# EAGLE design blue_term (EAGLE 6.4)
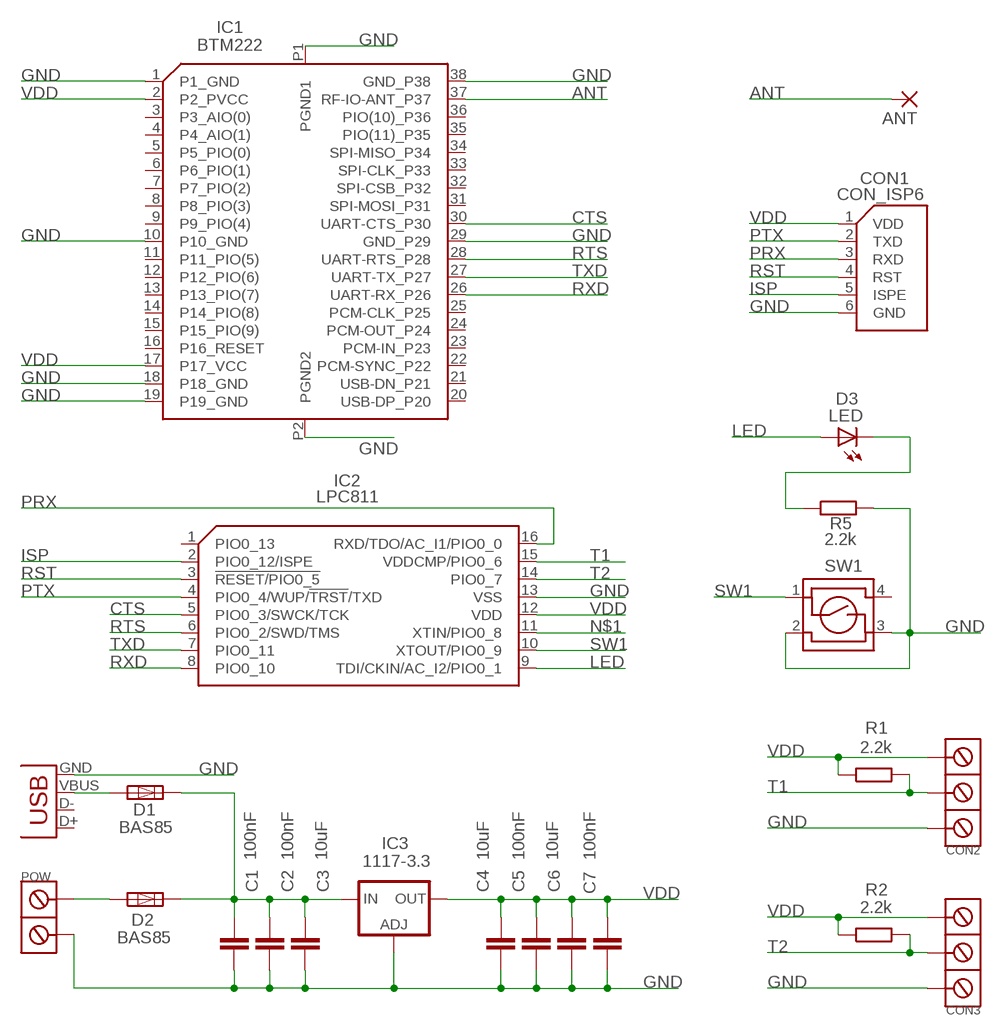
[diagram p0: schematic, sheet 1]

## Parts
ANT  2,54/1,0  [2,54/1,0]
C1  100nF  C-EUC1206  [C1206]
C2  100nF  C-EUC1206  [C1206]
C3  10uF  C-EUC1206  [C1206]
C4  10uF  C-EUC1206  [C1206]
C5  100nF  C-EUC1206  [C1206]
C6  10uF  C-EUC1206  [C1206]
C7  100nF  C-EUC1206  [C1206]
CON1  CON_ISP6  [CON6]
CON2  ARK3ARK3/500  [ARK3/500]
CON3  ARK3ARK3/500  [ARK3/500]
D1  BAS85  R-EU_R1206  [R1206]
D2  BAS85  R-EU_R1206  [R1206]
D3  LED  LEDCHIPLED_1206  [CHIPLED_1206]
IC1  BTM222  [BTM222]
IC2  LPC811  [TSSOP16]
IC3  1117-3.3  LM317MABDT  [DPACK]
POW  ARK2ARK2/500  [ARK2/500]
R1  2.2k  R-EU_R1206  [R1206]
R2  2.2k  R-EU_R1206  [R1206]
R5  2.2k  R-EU_R1206  [R1206]
SW1  6X6  [6X6]
USB  USB-MICROB  [USB-MICROB]

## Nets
ANT: ANT.1(P) IC1.37(RF-IO-ANT_P37)
CTS: IC1.30(UART-CTS_P30) IC2.5(PIO0_3/SWCK/TCK)
GND: C1.2 C2.2 C3.2 C4.2 C5.2 C6.2 C7.2 CON1.6(GND) CON2.1 CON3.1 IC1.1(P1_GND) IC1.10(P10_GND) IC1.18(P18_GND) IC1.19(P19_GND) IC1.29(GND_P29) IC1.38(GND_P38) IC1.P1(PGND1) IC1.P2(PGND2) IC2.13(VSS) IC3.1(ADJ) POW.2 R5.2 SW1.2 SW1.3 USB.GND
ISP: CON1.5(ISPE) IC2.2(PIO0_12/ISPE)
LED: D3.A IC2.9(TDI/CKIN/AC_I2/PIO0_1)
N$1: IC2.11(XTIN/PIO0_8)
N$2: D3.C R5.1
N$10: D1.1 USB.VBUS
N$11: C1.1 C2.1 C3.1 D1.2 D2.2 IC3.3(IN)
N$12: D2.1 POW.1
PRX: CON1.3(RXD) IC2.16(RXD/TDO/AC_I1/PIO0_0)
PTX: CON1.2(TXD) IC2.4(PIO0_4/WUP/!TRST!/TXD)
RST: CON1.4(RST) IC2.3(!RESET/PIO0_5)
RTS: IC1.28(UART-RTS_P28) IC2.6(PIO0_2/SWD/TMS)
RXD: IC1.26(UART-RX_P26) IC2.8(PIO0_10)
SW1: IC2.10(XTOUT/PIO0_9) SW1.1
T1: CON2.2 IC2.15(VDDCMP/PIO0_6) R1.2
T2: CON3.2 IC2.14(PIO0_7) R2.2
TXD: IC1.27(UART-TX_P27) IC2.7(PIO0_11)
VDD: C4.1 C5.1 C6.1 C7.1 CON1.1(VDD) CON2.3 CON3.3 IC1.2(P2_PVCC) IC1.17(P17_VCC) IC2.12(VDD) IC3.4(OUT) R1.1 R2.1
Unconnected: IC1.3(P3_AIO(0)) IC1.4(P4_AIO(1)) IC1.5(P5_PIO(0)) IC1.6(P6_PIO(1)) IC1.7(P7_PIO(2)) IC1.8(P8_PIO(3)) IC1.9(P9_PIO(4)) IC1.11(P11_PIO(5)) IC1.12(P12_PIO(6)) IC1.13(P13_PIO(7)) IC1.14(P14_PIO(8)) IC1.15(P15_PIO(9)) IC1.16(P16_RESET) IC1.20(USB-DP_P20) IC1.21(USB-DN_P21) IC1.22(PCM-SYNC_P22) IC1.23(PCM-IN_P23) IC1.24(PCM-OUT_P24) IC1.25(PCM-CLK_P25) IC1.31(SPI-MOSI_P31) IC1.32(SPI-CSB_P32) IC1.33(SPI-CLK_P33) IC1.34(SPI-MISO_P34) IC1.35(PIO(11)_P35) IC1.36(PIO(10)_P36) IC2.1(PIO0_13) SW1.4 USB.D+ USB.D-

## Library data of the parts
ANT = wirepad:2,54/1,0: THROUGH-HOLE PAD
C1-C7 = rcl:C-EU: CAPACITOR, European symbol
CON1 = LPC1114:CON_ISP6
CON2 CON3 = dimmer:ARK3
D1 D2 R1 R2 R5 = rcl:R-EU_: RESISTOR, European symbol
D3 = led:LED: LED
IC1 = BTM222:BTM222
IC2 = LPC8xx:LPC811
IC3 = v-reg:LM317?*: 500 mA Adjustable Output Positive Voltage Regulator Source: http://www.onsemi.co.jp .. LM317M-D.PDF
POW = dimmer:ARK2
SW1 = sw:6X6
USB = SparkFun:USB: USB Connectors USB-B-PTH is fully proven SKU : PRT-00139 USB-miniB is fully proven SKU : PRT-00587 USB-A-PCB is untested. USB-A-H is throughly reviewed, but untested. Spark Fun Electronics SKU : PRT-00437 USB-B-SMT is throughly reviewed, but untested. Needs silkscreen touching up. USB-A-S has not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

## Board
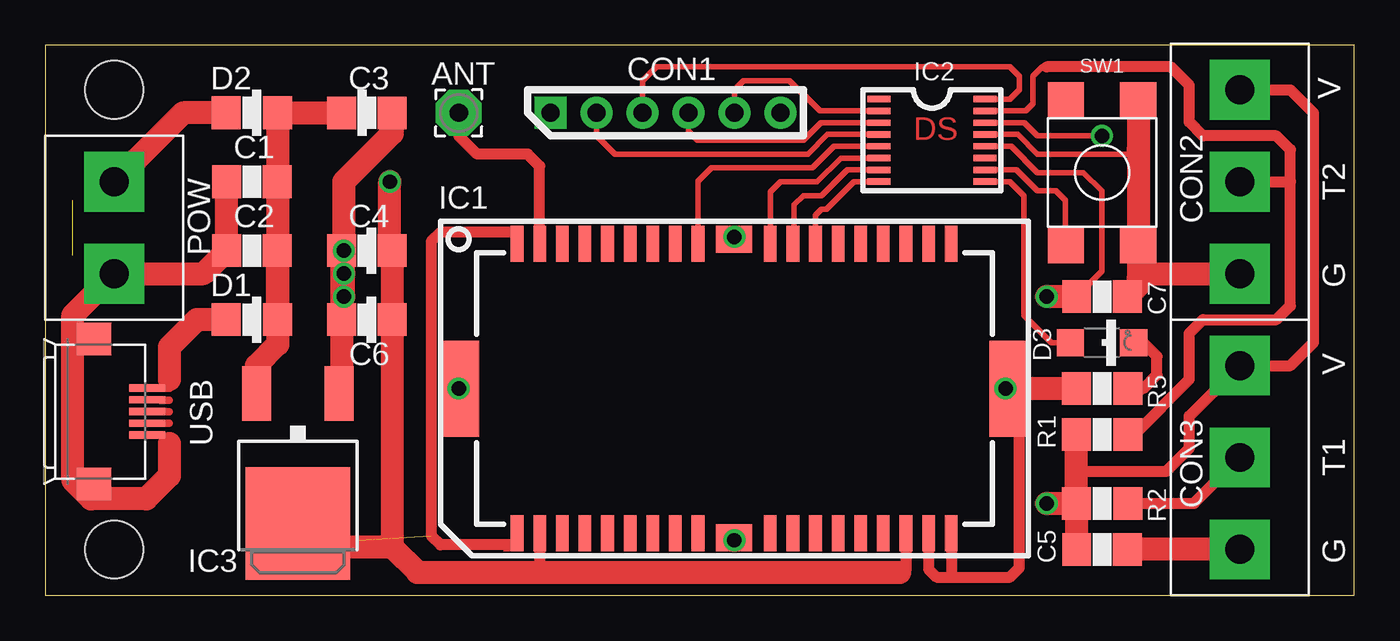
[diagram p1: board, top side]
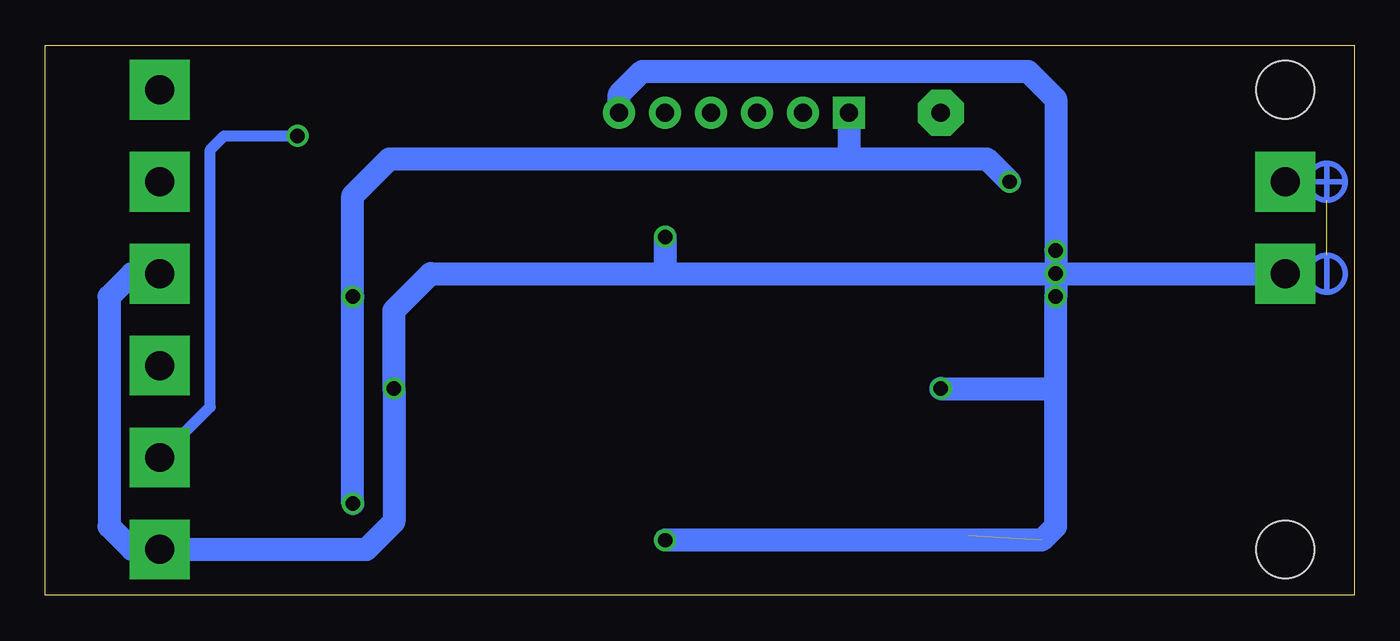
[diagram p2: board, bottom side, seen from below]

Size 72.37 x 30.4 mm. Coordinates in mm from the lower left corner, seen from the top.
Outline: 0,0 72.37,0 72.37,30.4 0,30.4 0,0
Copper layers (1*16): Top 0.035mm / dielectric 1.5mm / Bottom 0.035mm
Design rules "default": minimum track width 10mil, minimum drill 24mil, track to track 8mil, track to pad 8mil, pad to pad 8mil, via to via 8mil, smd to smd 8mil, copper to edge 40mil, drill to drill 8mil, minimum pad ring 10mil, minimum via ring 8mil, stop-mask expansion 4mil, vias tented up to drill 0mil, thermal gap 10mil
Holes 3.2 mm at 3.81,27.94 3.81,2.54

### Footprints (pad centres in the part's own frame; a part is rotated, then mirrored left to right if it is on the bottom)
2,54/1,0 = drill 1.016 pad 2.54 octagon: 1 0,0
C1206 = smd 1.6 x 1.8: 1 -1.4,0; 2 1.4,0
CON6 = drill 1 pad 1.778 square: 1 0,6.35 | drill 1 pad 1.778: 2 0,3.81; 3 0,1.27; 4 0,-1.27; 5 0,-3.81; 6 0,-6.35
ARK3/500 = drill 1.6 pad 3.302 square: 1 -5.08,0; 2 0,0; 3 5.08,0
R1206 = smd 1.6 x 1.803: 1 -1.422,0; 2 1.422,0
CHIPLED_1206 = smd 1.5 x 1.5: A 0,-1.75; C 0,1.75
BTM222 = smd 0.7 x 2: 1 -12.015,-8; 2 -10.765,-8; 3 -9.515,-8; 4 -8.265,-8; 5 -7.015,-8; 6 -5.765,-8; 7 -4.515,-8; 8 -3.265,-8; 9 -2.015,-8; 11 1.985,-8; 12 3.235,-8; 13 4.485,-8; 14 5.735,-8; 15 6.985,-8; 16 8.235,-8; 17 9.485,-8; 18 10.735,-8; 19 11.985,-8; 20 11.985,8; 21 10.735,8; 22 9.485,8; 23 8.235,8; 24 6.985,8; 25 5.735,8; 26 4.485,8; 27 3.235,8; 28 1.985,8; 30 -2.015,8; 31 -3.265,8; 32 -4.515,8; 33 -5.765,8; 34 -7.015,8; 35 -8.265,8; 36 -9.515,8; 37 -10.765,8; 38 -12.015,8 | smd 2 x 1.5: 10 -0.015,-8.25; 29 -0.015,8.25 | smd 2 x 5.3: P1 -15.115,0; P2 15.085,0
TSSOP16 = smd 0.356 x 1.27: 1 -2.275,-2.918; 2 -1.625,-2.918; 3 -0.975,-2.918; 4 -0.325,-2.918; 5 0.325,-2.918; 6 0.975,-2.918; 7 1.625,-2.918; 8 2.275,-2.918; 9 2.275,2.918; 10 1.625,2.918; 11 0.975,2.918; 12 0.325,2.918; 13 -0.325,2.918; 14 -0.975,2.918; 15 -1.625,2.918; 16 -2.275,2.918
DPACK = smd 1.6 x 3: 1 -2.28,-4.8; 3 2.28,-4.8 | smd 5.8 x 6.2: 4 0,2.38
ARK2/500 = drill 1.6 pad 3.302 square: 1 -2.54,0; 2 2.54,0
6X6 = smd 2 x 2: 1 -4,2; 2 -4,-2; 3 4,-2; 4 4,2
USB-MICROB = smd 0.4 x 2: D+ 0,3.1; D- -0.65,3.1; GND 1.3,3.1; ID 0.65,3.1; VBUS -1.3,3.1 | smd 1.8 x 1.9: GND@2 -4,0.15; GND@3 4,0.15

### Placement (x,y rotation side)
ANT  22.86,26.67 0 top
C1  11.43,22.86 180 top
C2  11.43,19.05 180 top
C3  17.78,26.67 0 top
C4  17.78,19.05 180 top
C5  58.42,2.54 0 top
C6  17.78,15.24 180 top
C7  58.42,16.51 0 top
CON1  34.29,26.67 90 top
CON2  66.04,22.86 90 top
CON3  66.04,7.62 90 top
D1  11.43,15.24 0 top
D2  11.43,26.67 0 top
D3  58.42,13.97 270 top
IC1  38.1,11.43 0 top
IC2  49.02,25.15 270 top
IC3  13.97,6.35 180 top
POW  3.81,20.32 270 top
R1  58.42,8.89 0 top
R2  58.42,5.08 0 top
R5  58.42,11.43 180 top
SW1  58.42,23.37 90 top
USB  2.54,10.16 270 top

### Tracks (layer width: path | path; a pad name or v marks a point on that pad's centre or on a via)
ANT
  Top 0.61: IC1.37 27.34,23.72 26.67,24.38 23.88,24.38 22.86,25.4 ANT.1
CTS
  Top 0.305: IC1.30 36.09,22.88 36.83,23.62 42.42,23.62 43.62,24.82 IC2.5
GND  (via drill 0.8)  (1 unrouted)
  Top 0.305: USB.GND 6.83,8.86 6.86,8.89 6.86,8.38 | IC2.13 53.78,25.47 54.86,24.38 60.17,24.38 60.42,24.64
  Top 0.61: IC1.38 26.09,19.99 26.16,20.07 21.84,20.07 21.34,19.56 21.34,3.3 21.84,2.79 25.91,2.79 26.09,2.97 IC1.1 | IC1.18 48.84,1.46 49.28,1.02 50.29,1.02 | 50.29,1.02 53.34,1.02 53.85,1.52 53.85,10.77 IC1.P2 | IC1.19 50.09,1.22 50.29,1.02
  Top 1.27: C4.2 C6.2 16.38,11.28 IC3.1 | C1.2 C2.2 8.76,17.78 POW.2 1.52,15.49 1.52,6.35 2.54,5.33 5.59,5.33 6.86,6.6 6.86,8.38 | v16.51,19.05 C4.2 | CON3.1 C5.2 | C3.2 19.18,25.53 16.51,22.86 v16.51,19.05 | SW1.3 60.42,24.64 SW1.2 60.42,17.53 | 60.42,17.53 60.42,17.11 C7.2 | 60.42,17.53 60.67,17.78 CON2.1 | R5.2 IC1.P2 v53.09,11.43 | v16.51,16.51 v16.51,17.78 v16.51,19.05 | v16.51,19.05 16.51,19.18 C4.2 | IC1.29 38.09,19.8 v38.1,19.81 | IC1.10 38.09,3.03 v38.1,3.05 | IC1.P1 v22.86,11.43
  Bottom 1.27: CON2.1 67.56,17.78 68.83,16.51 68.83,3.81 67.56,2.54 CON3.1 54.61,2.54 53.09,4.06 v53.09,11.43 53.09,15.75 51.05,17.78 37.85,17.78 | 37.85,17.78 v16.51,17.78 | CON1.6 40.64,27.69 39.37,28.96 18.03,28.96 16.51,27.43 v16.51,19.05 v16.51,17.78 | v16.51,17.78 POW.2 | v16.51,17.78 v16.51,16.51 16.51,11.68 | v38.1,19.81 38.1,18.03 37.85,17.78 | 16.51,11.68 16.51,3.81 17.27,3.05 v38.1,3.05 | v22.86,11.43 16.76,11.43 16.51,11.68
ISP
  Top 0.305: IC2.2 42.83,26.77 41.15,28.45 38.61,28.45 38.1,27.94 CON1.5
LED
  Top 0.305: 56.39,13.97 55.63,13.97 54.1,15.49 54.1,22.1 53.34,22.86 51.95,22.86 IC2.9
  Top 0.61: D3.A 56.39,13.97
N$2
  Top 0.61: R5.1 60.71,11.43 61.47,12.19 61.47,13.21 60.71,13.97 D3.C
N$3
  Top 0.406: 6.35,10.79 6.86,10.79
N$4
  Top 0.406: 6.48,10.16 6.86,10.16
N$5
  Top 0.406: 6.35,9.52 6.86,9.52
N$6  (1 unrouted)
  Bottom 0.305: 1.52,23.88 1.52,21.84 | 1.52,18.8 1.52,16.76
N$7
  Bottom 0.305: 0.51,22.86 2.54,22.86
N$10
  Top 0.305: 6.89,11.46 6.89,12.67 6.86,11.94
  Top 0.406: USB.VBUS 6.89,11.46
  Top 1.27: D1.1 8.38,15.24 6.86,13.72 6.86,11.94
N$11
  Top 1.27: 12.85,22.86 D2.2 C3.1 | 12.85,22.86 12.85,19.05 | 12.85,19.05 D1.2 | C1.1 12.85,22.86 | 12.85,19.05 C2.1 12.83,15.26 D1.2 | D1.2 12.85,13.87 11.68,12.7 IC3.3
N$12
  Top 1.27: D2.1 7.62,26.67 POW.1
PRX
  Top 0.305: IC2.16 53.33,27.42 53.85,27.94 53.85,28.7 53.34,29.21 33.78,29.21 33.02,28.45 CON1.3
PTX
  Top 0.305: IC2.4 43.25,25.47 42.16,24.38 31.5,24.38 30.48,25.4 CON1.2
RST
  Top 0.305: IC2.3 42.88,26.12 41.91,25.15 36.07,25.15 35.56,25.65 CON1.4
RTS
  Top 0.305: IC1.28 40.09,22.31 40.64,22.86 42.67,22.86 43.98,24.17 IC2.6
RXD
  Top 0.305: IC2.8 44.72,22.87 43.18,21.34 42.93,21.34 42.59,21 IC1.26
SW1
  Top 0.305: IC2.10 53.7,23.52 54.86,22.35 55.88,22.35 56.39,21.84 56.39,19.4 SW1.1
T1
  Top 0.305: 55.37,29.21 55.12,29.21 54.61,28.7 54.61,27.18 54.2,26.77 IC2.15
  Top 0.61: 55.37,29.21 62.23,29.21 63.25,28.19 63.25,26.16 64.01,25.4 68.07,25.4 68.83,24.64 68.83,22.86 | R1.2 60.2,8.89 63.25,11.94 63.25,14.48 64.01,15.24 68.07,15.24 68.83,16 68.83,22.86 | CON2.2 68.83,22.86
T2  (via drill 0.8)
  Top 0.305: IC2.14 54.14,26.12 54.86,25.4 v58.42,25.4
  Top 0.61: R2.2 63.5,5.08 CON3.2
  Bottom 0.61: CON3.2 63.25,10.41 63.25,24.64 62.48,25.4 v58.42,25.4
TXD
  Top 0.305: IC2.7 44.35,23.52 42.93,22.1 41.91,22.1 41.4,21.59 41.4,19.5 IC1.27
VDD  (via drill 0.8)
  Top 0.305: IC2.12 53.41,24.82 54.86,23.37 57.4,23.37 58.42,22.35 58.42,17.91 C7.1
  Top 0.61: IC1.2 27.34,1.37 27.43,1.27 | IC1.17 47.59,1.44 47.24,1.27 | 57,6.86 61.98,6.86 63.25,8.13 63.25,9.91 CON3.3 68.83,12.7 70.1,13.97 70.1,26.67 68.83,27.94 CON2.3
  Top 1.27: 19.18,2.66 C6.1 19.18,18.92 | 19.18,2.66 20.57,1.27 27.43,1.27 47.24,1.27 | R2.1 57,2.56 C5.1 57.02,4.95 57.15,5.08 | 19.18,2.66 15.11,2.66 14.73,2.29 14.73,3.21 IC3.4 | R2.1 57,6.86 R1.1 | C7.1 v55.37,16.51 | v55.37,5.08 R2.1 | C4.1 19.18,18.92 | 19.18,18.92 19.05,19.05 v19.05,22.86
  Bottom 1.27: 27.94,24.13 53.34,24.13 55.37,22.1 v55.37,16.51 v55.37,5.08 | 27.94,24.13 20.32,24.13 v19.05,22.86 | CON1.1 27.94,24.13
(copper drawn outside any net)
  shapes: Bottom circle x2

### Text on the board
Top: DS
tPlace: V | T2 | G | V | T1 | G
